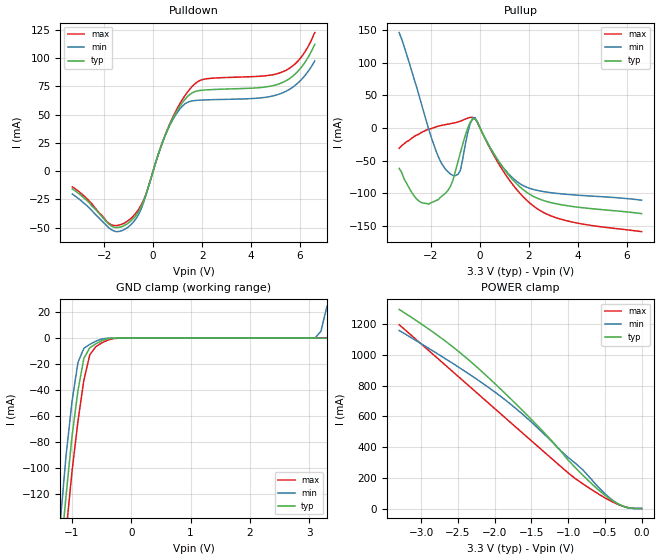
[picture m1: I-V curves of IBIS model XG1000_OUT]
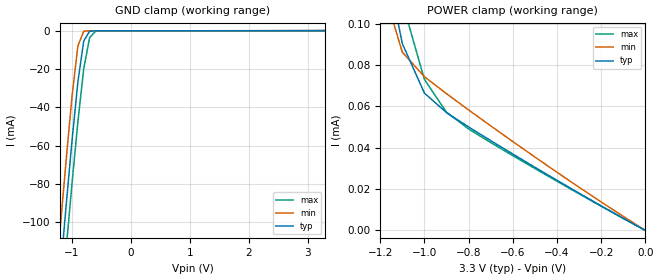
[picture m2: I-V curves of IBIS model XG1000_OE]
|   IBIS File xg1kcb-c.ibs
|   Epson Toyocom Corporation , 2005
[IBIS Ver]   2.1
[Comment Char]   |_char
[File name]   xg1kcb-c.ibs
[File Rev]   2.0
[Date]   2006/12/26
[Source]
[Notes]
[Disclaimer]
This information is for modeling purposes only, and is not guaranteed.
Property of Epson Toyocom Corp.,
unauthorized reproduction and/or distribution is strictly prohibited.
[Copyright]
Copyright 2005, Epson Toyocom Corp.
|   Component XG-1000CB_C
[Component]   XG-1000CB_C
[Manufacturer]   Epson Toyocom Corp.
[Package]
| variable   typ   min   max
R_pkg   0.583   NA   NA
L_pkg   1.35nH   NA   NA
C_pkg   1.70pF   NA   NA
[Pin]signal_name   model_name   R_pin   L_pin   C_pin
1   oe   XG1000_OE   NA   NA   NA
2   vss   GND   NA   NA   NA
3   out   XG1000_OUT   NA   NA   NA
4   vdd   POWER   NA   NA   NA
| Models and submodels in the file (2): XG1000_OUT (3-state), XG1000_OE (Input)
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|   Model XG1000_OUT
[Model]   XG1000_OUT
Model_type 3-state
Enable Active-High
Polarity Inverting
C_comp   3p   2.5p   3.5p
[Temperature Range] 25   -40   85
[Voltage Range]   3.3   3.0   3.6
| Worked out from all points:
|   slope of the pulldown table from 0 to 0.495 V, typ, clamps not added: 15.6 ohm
|   slope of the pullup table from 0 to 0.495 V, typ, clamps not added: 14.1 ohm
|   GND clamp passes 1 mA (typ) near -0.43 V on its own axis
|   POWER clamp passes 1 mA (typ) near -0.11 V on its own axis
[Pullup]
-3.3V     -62.09mA   146.3mA    -31.24mA
-2.8V     -98.11mA   88.85mA    -16.17mA
-2.4V     -114.3mA   37.98mA    -7.254mA
-1.7V     -109.8mA   -44.13mA   2.662mA
-1.2V     -89.47mA   -70.82mA   6.55mA
-800mV    -38.13mA   -65.09mA   10.38mA
-400mV    8.472mA    6.607mA    16.22mA
-200mV    13.71mA    15.93mA    13.91mA
1V        -63.98mA   -63.13mA   -69.07mA
2.3V      -107.1mA   -95.48mA   -123mA
3.7V      -120.1mA   -102.3mA   -143.8mA
6.6V      -131.4mA   -110.9mA   -159.1mA
[Pulldown]
-3.3V     -15.76mA   -20.26mA   -13.85mA
-1.8V     -47.02mA   -50.27mA   -46.3mA
-1.1V     -47.19mA   -50.68mA   -45mA
-700mV    -39.17mA   -42.09mA   -37.05mA
-400mV    -27.43mA   -28.39mA   -26.24mA
400mV     26.38mA    26.45mA    26.48mA
800mV     46.3mA     45.29mA    47.42mA
1.2V      60.65mA    57.52mA    63.45mA
2V        71.48mA    62.8mA     80.77mA
5.3V      78.49mA    69.31mA    87.82mA
6V        90.32mA    79.67mA    99.43mA
6.6V      112mA      97.37mA    122.5mA
[GND Clamp]
-3.3V     -1.228A    -1.271A    -1.212A
-1.2V     -170.3mA   -142.5mA   -196.7mA
-1.1V     -120.7mA   -89.99mA   -148.9mA
-1V       -75.55mA   -48.78mA   -102.4mA
-900mV    -40.37mA   -18.72mA   -63.95mA
-800mV    -15.58mA   -7.854mA   -32.35mA
-700mV    -7.457mA   -4.83mA    -12.88mA
-500mV    -2.099mA   -692uA     -3.749mA
-200mV    -1.934uA   -15.85nA   -32.95uA
3.1V      985.2pA    240.6nA    -129.1nA
3.2V      1.672nA    5.264mA    -96.22nA
3.3V      5.855nA    24.33mA    -62.21nA
[POWER Clamp]
-3.3V     1.296A     1.16A      1.197A
-2.7V     1.1A       984.2mA    945.5mA
-2.2V     902.8mA    827.5mA    735.1mA
-1.7V     675.5mA    646.7mA    524.7mA
-1.3V     480.6mA    472mA      356.9mA
-1.1V     373.6mA    376mA      273.4mA
-900mV    264.9mA    293.8mA    194mA
-800mV    217mA      251.7mA    160.9mA
-600mV    126.5mA    144.8mA    98.33mA
-400mV    51.62mA    55.26mA    43.48mA
-200mV    6.958mA    5.264mA    7.215mA
0V        5.855nA    12.4pA     351.5nA
[Ramp]
R_load=50
dV/dt_r   1.103E+0/1.198E-10   1.042E+0/8.584E-11   1.190E+0/7.697E-11
dV/dt_f   1.076E+0/7.420E-11   1.011E+0/1.171E-10   1.145E+0/1.161E-10
|   Model XG1000_OE
[Model]   XG1000_OE
Model_type Input
Vinh=2.31
Vinl=0.99
C_comp   3p   2.5p   3.5p
[Temperature Range] 25   -40   85
[Voltage Range]   3.3   3.0   3.6
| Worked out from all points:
|   GND clamp passes 1 mA (typ) near -0.71 V on its own axis
|   POWER clamp passes 1 mA (typ) near -2.16 V on its own axis
[GND Clamp]
-3.3V     -919.3mA   -898.4mA   -939.8mA
-1.3V     -163.5mA   -139.9mA   -186.2mA
-1.2V     -127.3mA   -103.6mA   -150.1mA
-1.1V     -91.93mA   -68.17mA   -114.7mA
-1V       -57.91mA   -34.82mA   -80.28mA
-900mV    -26.98mA   -8.136mA   -47.86mA
-800mV    -5.454mA   -302uA     -19.91mA
-700mV    -354.8uA   -80.39uA   -3.645mA
-600mV    -85.43uA   -78.8uA    -361.6uA
3.3V      3.297pA    20.89uA    -16.39uA
[POWER Clamp]
-3.3V     2.11mA     2.096mA    2.129mA
-1.2V     143.2uA    122.1uA    171.1uA
-1.1V     90.42uA    86.25uA    110.5uA
-1V       66.44uA    74.36uA    73.06uA
-900mV    57.01uA    66.16uA    57.16uA
-800mV    50.06uA    58.3uA     49.09uA
-700mV    43.46uA    50.59uA    42.51uA
-300mV    18.01uA    20.89uA    17.72uA
0V        3.24pA     2.874pA    4.54pA
